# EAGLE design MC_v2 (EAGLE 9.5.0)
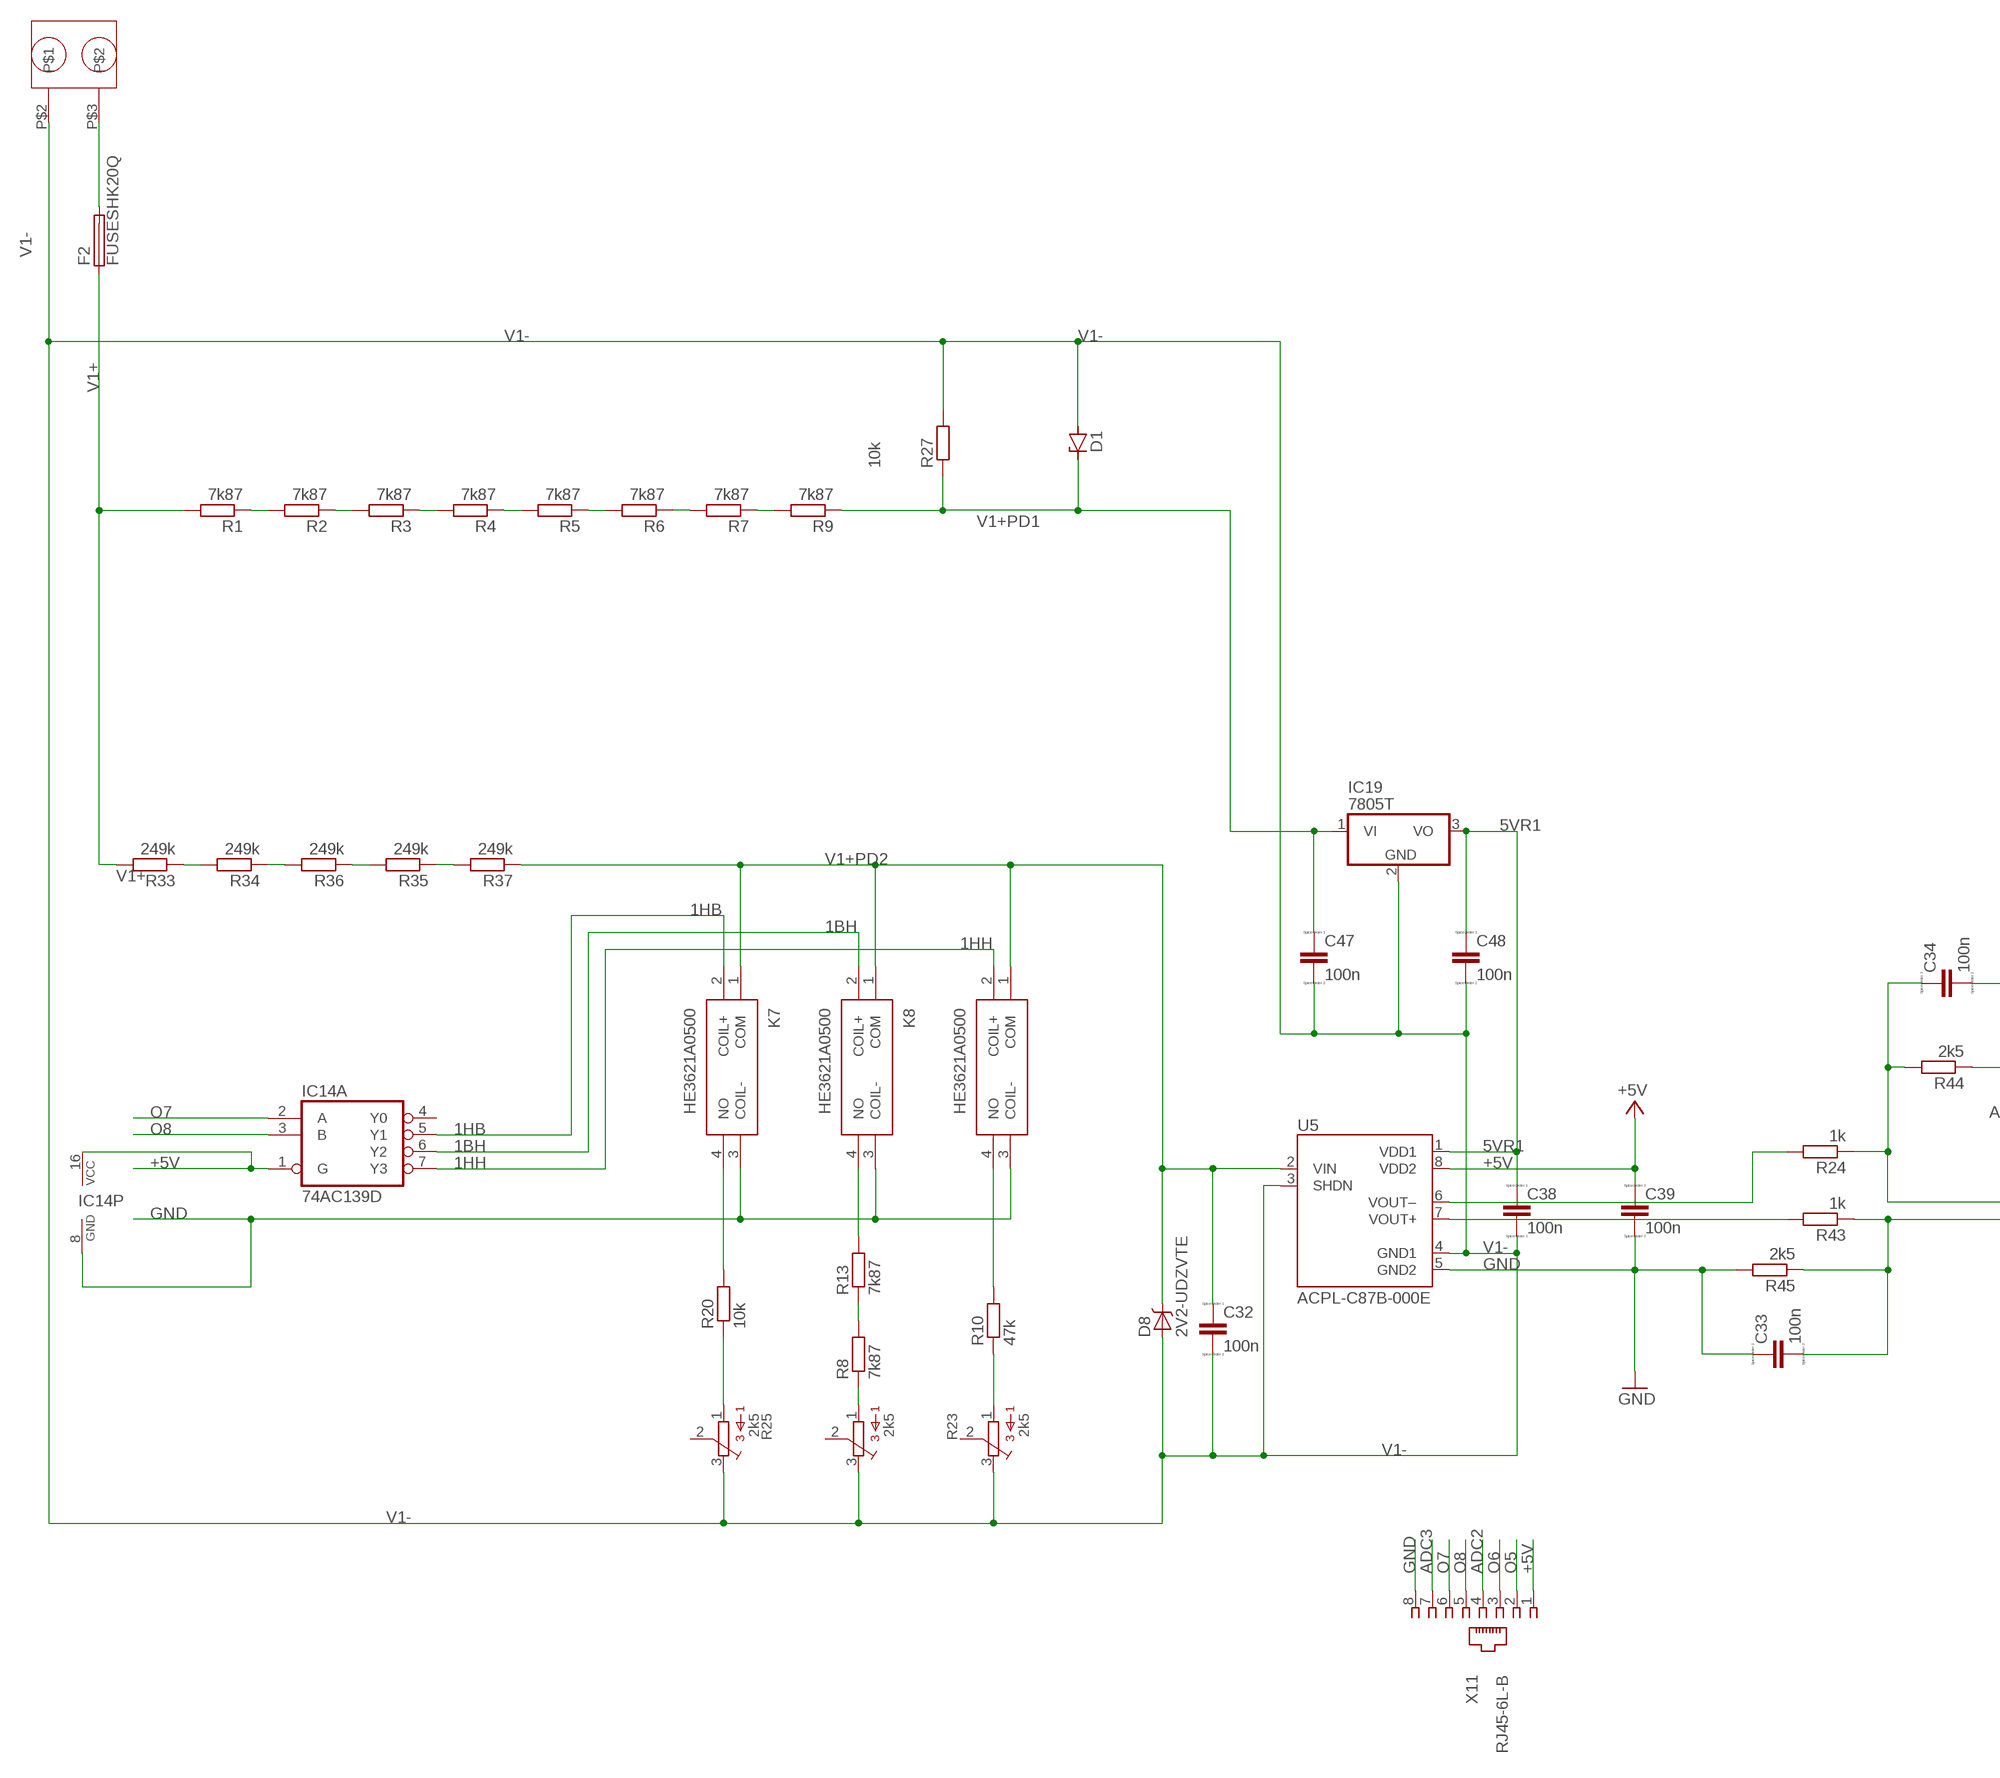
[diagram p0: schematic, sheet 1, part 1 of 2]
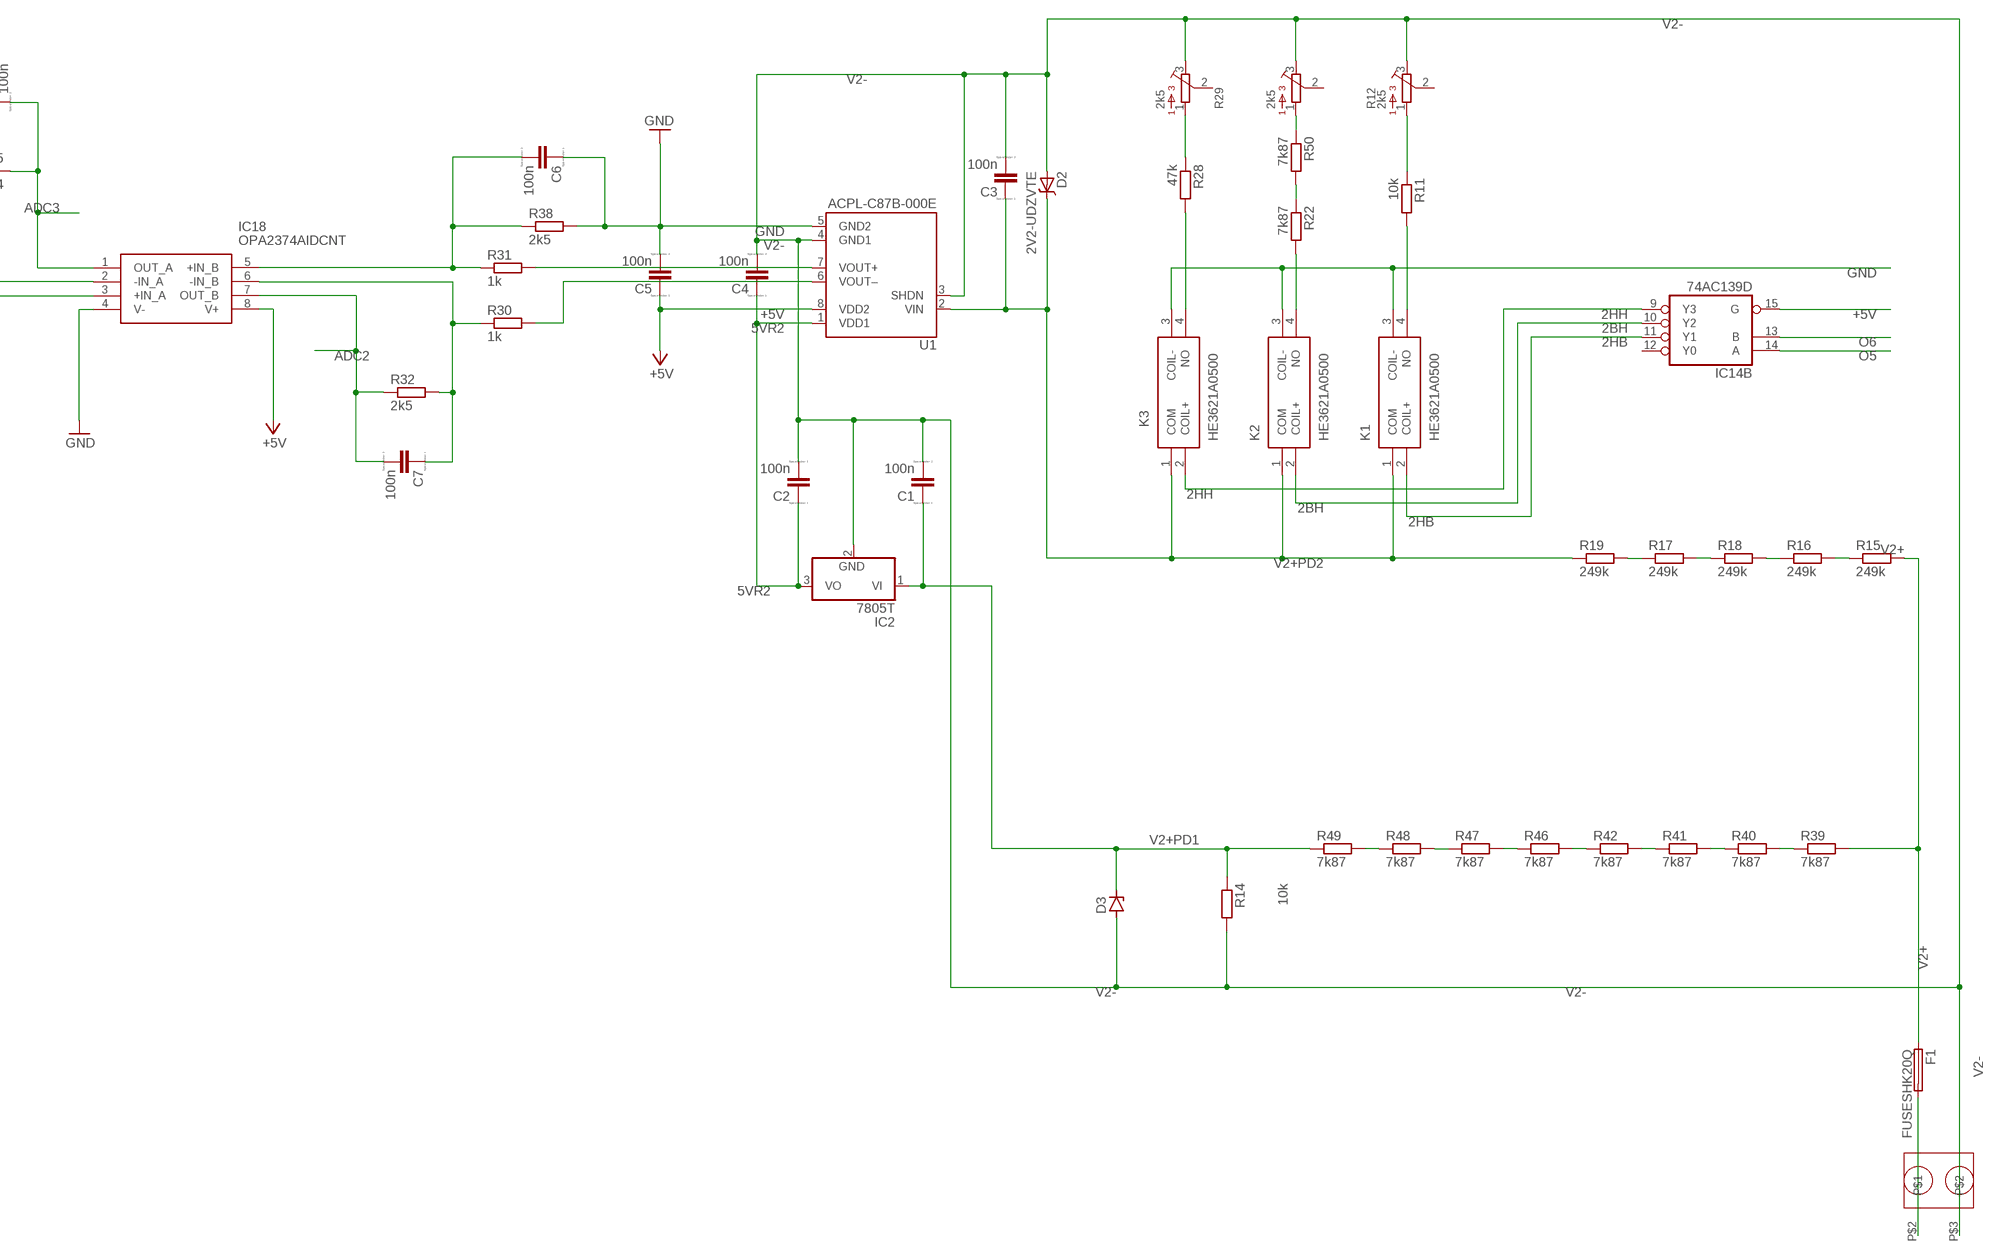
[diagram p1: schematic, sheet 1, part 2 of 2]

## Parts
C1  100n  CC2012  [C2012]
C2  100n  CC2012  [C2012]
C3  100n  CC2012  [C2012]
C4  100n  CC2012  [C2012]
C5  100n  CC2012  [C2012]
C6  100n  CC2012  [C2012]
C7  100n  CC2012  [C2012]
C32  100n  CC2012  [C2012]
C33  100n  CC2012  [C2012]
C34  100n  CC2012  [C2012]
C38  100n  CC2012  [C2012]
C39  100n  CC2012  [C2012]
C47  100n  CC2012  [C2012]
C48  100n  CC2012  [C2012]
D1  ZENER-DIODEDO41Z10  [DO41Z10]
D2  2V2-UDZVTE  BAS70J  [SOD-323]
D3  ZENER-DIODEDO41Z10  [DO41Z10]
D8  2V2-UDZVTE  BAS70J  [SOD-323]
F1  FUSESHK20Q  [SHK20Q]
F2  FUSESHK20Q  [SHK20Q]
IC2  7805T  [TO220H]
IC14  74AC139D  [SO16]
IC18  OPA2374AIDCNT  [SOT65P280X145-8N]
IC19  7805T  [TO220H]
K1  HE3621A0500  [HE3621A0500]
K2  HE3621A0500  [HE3621A0500]
K3  HE3621A0500  [HE3621A0500]
K7  HE3621A0500  [HE3621A0500]
K8  HE3621A0500  [HE3621A0500]
K9  HE3621A0500  [HE3621A0500]
R1  7k87  R-EU_M0805  [M0805]
R2  7k87  R-EU_M0805  [M0805]
R3  7k87  R-EU_M0805  [M0805]
R4  7k87  R-EU_M0805  [M0805]
R5  7k87  R-EU_M0805  [M0805]
R6  7k87  R-EU_M0805  [M0805]
R7  7k87  R-EU_M0805  [M0805]
R8  7k87  R-EU_M0805  [M0805]
R9  7k87  R-EU_M0805  [M0805]
R10  47k  R-EU_M0805  [M0805]
R11  10k  R-EU_M0805  [M0805]
R12  2k5  3362P  [3362P]
R13  7k87  R-EU_M0805  [M0805]
R14  10k  R-EU_M0805  [M0805]
R15  249k  R-EU_M0805  [M0805]
R16  249k  R-EU_M0805  [M0805]
R17  249k  R-EU_M0805  [M0805]
R18  249k  R-EU_M0805  [M0805]
R19  249k  R-EU_M0805  [M0805]
R20  10k  R-EU_M0805  [M0805]
R21  2k5  3362P  [3362P]
R22  7k87  R-EU_M0805  [M0805]
R23  2k5  3362P  [3362P]
R24  1k  R-EU_M0805  [M0805]
R25  2k5  3362P  [3362P]
R26  2k5  3362P  [3362P]
R27  10k  R-EU_M0805  [M0805]
R28  47k  R-EU_M0805  [M0805]
R29  2k5  3362P  [3362P]
R30  1k  R-EU_M0805  [M0805]
R31  1k  R-EU_M0805  [M0805]
R32  2k5  R-EU_M0805  [M0805]
R33  249k  R-EU_M0805  [M0805]
R34  249k  R-EU_M0805  [M0805]
R35  249k  R-EU_M0805  [M0805]
R36  249k  R-EU_M0805  [M0805]
R37  249k  R-EU_M0805  [M0805]
R38  2k5  R-EU_M0805  [M0805]
R39  7k87  R-EU_M0805  [M0805]
R40  7k87  R-EU_M0805  [M0805]
R41  7k87  R-EU_M0805  [M0805]
R42  7k87  R-EU_M0805  [M0805]
R43  1k  R-EU_M0805  [M0805]
R44  2k5  R-EU_M0805  [M0805]
R45  2k5  R-EU_M0805  [M0805]
R46  7k87  R-EU_M0805  [M0805]
R47  7k87  R-EU_M0805  [M0805]
R48  7k87  R-EU_M0805  [M0805]
R49  7k87  R-EU_M0805  [M0805]
R50  7k87  R-EU_M0805  [M0805]
U1  ACPL-C87B-000E  [SOIC127P1150X360-8N]
U5  ACPL-C87B-000E  [SOIC127P1150X360-8N]
U$1  BORNIER-508  [BORNIER-508_FOOTPRINT]
U$20  BORNIER-508  [BORNIER-508_FOOTPRINT]
X11  RJ45-6L-B  [RJ45-NO-SHIELD]

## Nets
1BH: IC14.6(A:Y2) K8.2(COIL+)
1HB: IC14.5(A:Y1) K7.2(COIL+)
1HH: IC14.7(A:Y3) K9.2(COIL+)
2BH: IC14.10(B:Y2) K2.2(COIL+)
2HB: IC14.11(B:Y1) K1.2(COIL+)
2HH: IC14.9(B:Y3) K3.2(COIL+)
5VR1: C38.1 C48.1 IC19.3(VO) U5.1(VDD1)
5VR2: C2.1 C4.1 IC2.3(VO) U1.1(VDD1)
+5V [power]: C5.1 C39.1 IC14.1(A:G) IC14.15(B:G) IC14.16(P:VCC) IC18.8(V+) U1.8(VDD2) U5.8(VDD2) X11.1
ADC2: C7.2 IC18.7(OUT_B) R32.1 X11.4
ADC3: C34.2 IC18.1(OUT_A) R44.1 X11.7
GND: C5.2 C6.1 C33.1 C39.2 IC14.8(P:GND) IC18.4(V-) K1.3(COIL-) K2.3(COIL-) K3.3(COIL-) K7.3(COIL-) K8.3(COIL-) K9.3(COIL-) R38.2 R45.2 U1.5(GND2) U5.5(GND2) X11.8
N$1: F1.2A U$1.P$2
N$2: F2.2A U$20.P$3
N$3: R8.1 R21.1
N$4: R8.2 R13.1
N$5: R34.1 R36.2
N$6: R1.1 R2.2
N$7: R2.1 R3.2
N$8: R3.1 R4.2
N$9: R4.1 R5.2
N$10: R5.1 R6.2
N$11: R6.1 R7.2
N$12: R7.1 R9.2
N$13: K7.4(NO) R20.2
N$14: R35.1 R37.2
N$15: R10.1 R23.1
N$16: C6.2 IC18.5(+IN_B) R31.1 R38.1
N$17: R17.2 R18.1
N$18: K9.4(NO) R10.2
N$19: R15.1 R16.2
N$20: R31.2 U1.7(VOUT+)
N$21: R30.2 U1.6(VOUT–)
N$22: C7.1 IC18.6(-IN_B) R30.1 R32.2
N$23: R11.1 R12.1
N$24: K1.4(NO) R11.2
N$25: K2.4(NO) R22.2
N$26: K3.4(NO) R28.2
N$27: R28.1 R29.1
N$30: R26.1 R50.1
N$31: R22.1 R50.2
N$32: R39.1 R40.2
N$33: R40.1 R41.2
N$34: R41.1 R42.2
N$35: R42.1 R46.2
N$36: R46.1 R47.2
N$37: R47.1 R48.2
N$38: R48.1 R49.2
N$39: R16.1 R18.2
N$40: R17.1 R19.2
N$58: R20.1 R25.1
N$69: C33.2 IC18.3(+IN_A) R43.1 R45.1
N$73: R35.2 R36.1
N$74: R33.1 R34.2
N$82: R43.2 U5.7(VOUT+)
N$83: R24.2 U5.6(VOUT–)
N$84: C34.1 IC18.2(-IN_A) R24.1 R44.2
N$107: K8.4(NO) R13.2
O5: IC14.14(B:A) X11.2
O6: IC14.13(B:B) X11.3
O7: IC14.2(A:A) X11.6
O8: IC14.3(A:B) X11.5
V1+: F2.1A R1.2 R33.2
V1+PD1: C47.1 D1.C IC19.1(VI) R9.1 R27.1
V1+PD2: C32.1 D8.C K7.1(COM) K8.1(COM) K9.1(COM) R37.1 U5.2(VIN)
V1-: C32.2 C38.2 C47.2 C48.2 D1.A D8.A IC19.2(GND) R21.3 R23.3 R25.3 R27.2 U5.3(SHDN) U5.4(GND1) U$20.P$2
V2+: F1.1A R15.2 R39.2
V2+PD1: C1.1 D3.C IC2.1(VI) R14.1 R49.1
V2+PD2: C3.1 D2.C K1.1(COM) K2.1(COM) K3.1(COM) R19.1 U1.2(VIN)
V2-: C1.2 C2.2 C3.2 C4.2 D2.A D3.A IC2.2(GND) R12.3 R14.2 R26.3 R29.3 U1.3(SHDN) U1.4(GND1) U$1.P$3
Unconnected: IC14.4(A:Y0) IC14.12(B:Y0) R12.2 R21.2 R23.2 R25.2 R26.2 R29.2

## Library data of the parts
C1-C7 C32-C34 C38 C39 C47 C48 = eagle-ltspice:C: CAPACITOR, European symbol; SPICEMODEL: NONE; SPICEPREFIX: C
D1 D3 = diode:ZENER-DIODE: Z-Diode
D2 D8 = ELL-i-DiscreteSemi:BAS70: Silicon Schottky Diodes
F1 F2 = fuse:FUSE: Fuse; OC_FARNELL: unknown; OC_NEWARK: unknown
IC2 IC19 = linear:78*: Positive VOLTAGE REGULATOR Source: http://cache.national.com/ds/LM/LM78L05.pdf http://www.fairchildsemi.com/ds/LM/LM7805.pdf
IC14 = 74xx-eu:74*139: Dual 2-line to 4-line DECODER/DEMULTIPLEXER; SPICEPREFIX: I
IC18 = OPA2374AIDCNT:OPA2374AIDCNT: Texas Instruments OPA2374AIDCNT, Dual Op Amp, 6.5MHz CMOS, Rail to Rail, 3 V, 5 V, 8-Pin SOT-23 Source: Datasheet; DESCRIPTION: Texas Instruments OPA2374AIDCNT, Dual Op Amp, 6.5MHz CMOS, Rail to Rail, 3 V, 5 V, 8-Pin SOT-23; HEIGHT: mm; MANUFACTURER_NAME: Texas Instruments; MANUFACTURER_PART_NUMBER: OPA2374AIDCNT; MOUSER_PART_NUMBER: 595-OPA2374AIDCNT; MOUSER_PRICE-STOCK: https://www.mouser.com/Search/Refine.aspx?Keyword=595-OPA2374AIDCNT
K1-K3 K7-K9 = HE3621A0500:HE3621A0500: Reed Relays REED RELAY Source: Datasheet; DESCRIPTION: Reed Relays REED RELAY; HEIGHT: 7mm; MANUFACTURER_NAME: Hamlin / Littelfuse; MANUFACTURER_PART_NUMBER: HE3621A0500; MOUSER_PART_NUMBER: 934-HE3621A0500; MOUSER_PRICE-STOCK: https://www.mouser.com/Search/Refine.aspx?Keyword=934-HE3621A0500
R1-R11 R13-R20 R22 R24 R27 R28 R30-R50 = rcl:R-EU_: RESISTOR, European symbol; SPICEPREFIX: R
R12 R21 R23 R25 R26 R29 = bourns:3362: 3362 Series 1/4" Square Trimmer
U1 U5 = ACPL-C87B-000E:ACPL-C87B-000E: Precision Optically Isolated Voltage Sensor; AVAILABILITY: Unavailable; DESCRIPTION: Isolation Amplifier, Optically, 1, 9.9 mV, 5 kV, 3V to 5.5V, SOIC, 8; MF: Broadcom Limited; MP: ACPL-C87B-000E; PACKAGE: SO-8 Broadcom; PRICE: None
U$1 U$20 = bornier-508:BORNIER-508
X11 = con-tycoelectronics:RJ45: CORCOM Modular RJ Jacks No Shield Source: www.tycoelectronics.com .. ENG_DS_1654001_1099_RJ_L_0507.pdf; MPN: RJ45-6L-B; OC_FARNELL: unknown; OC_NEWARK: 16R6090

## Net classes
0 default: width 0.152 mm, drill 0.61 mm, clearance 0.152 mm
1 power: width 0.152 mm, drill 0.61 mm, clearance 0.152 mm
2 VIN: width 0.61 mm, drill 0.61 mm, clearance 0.254 mm

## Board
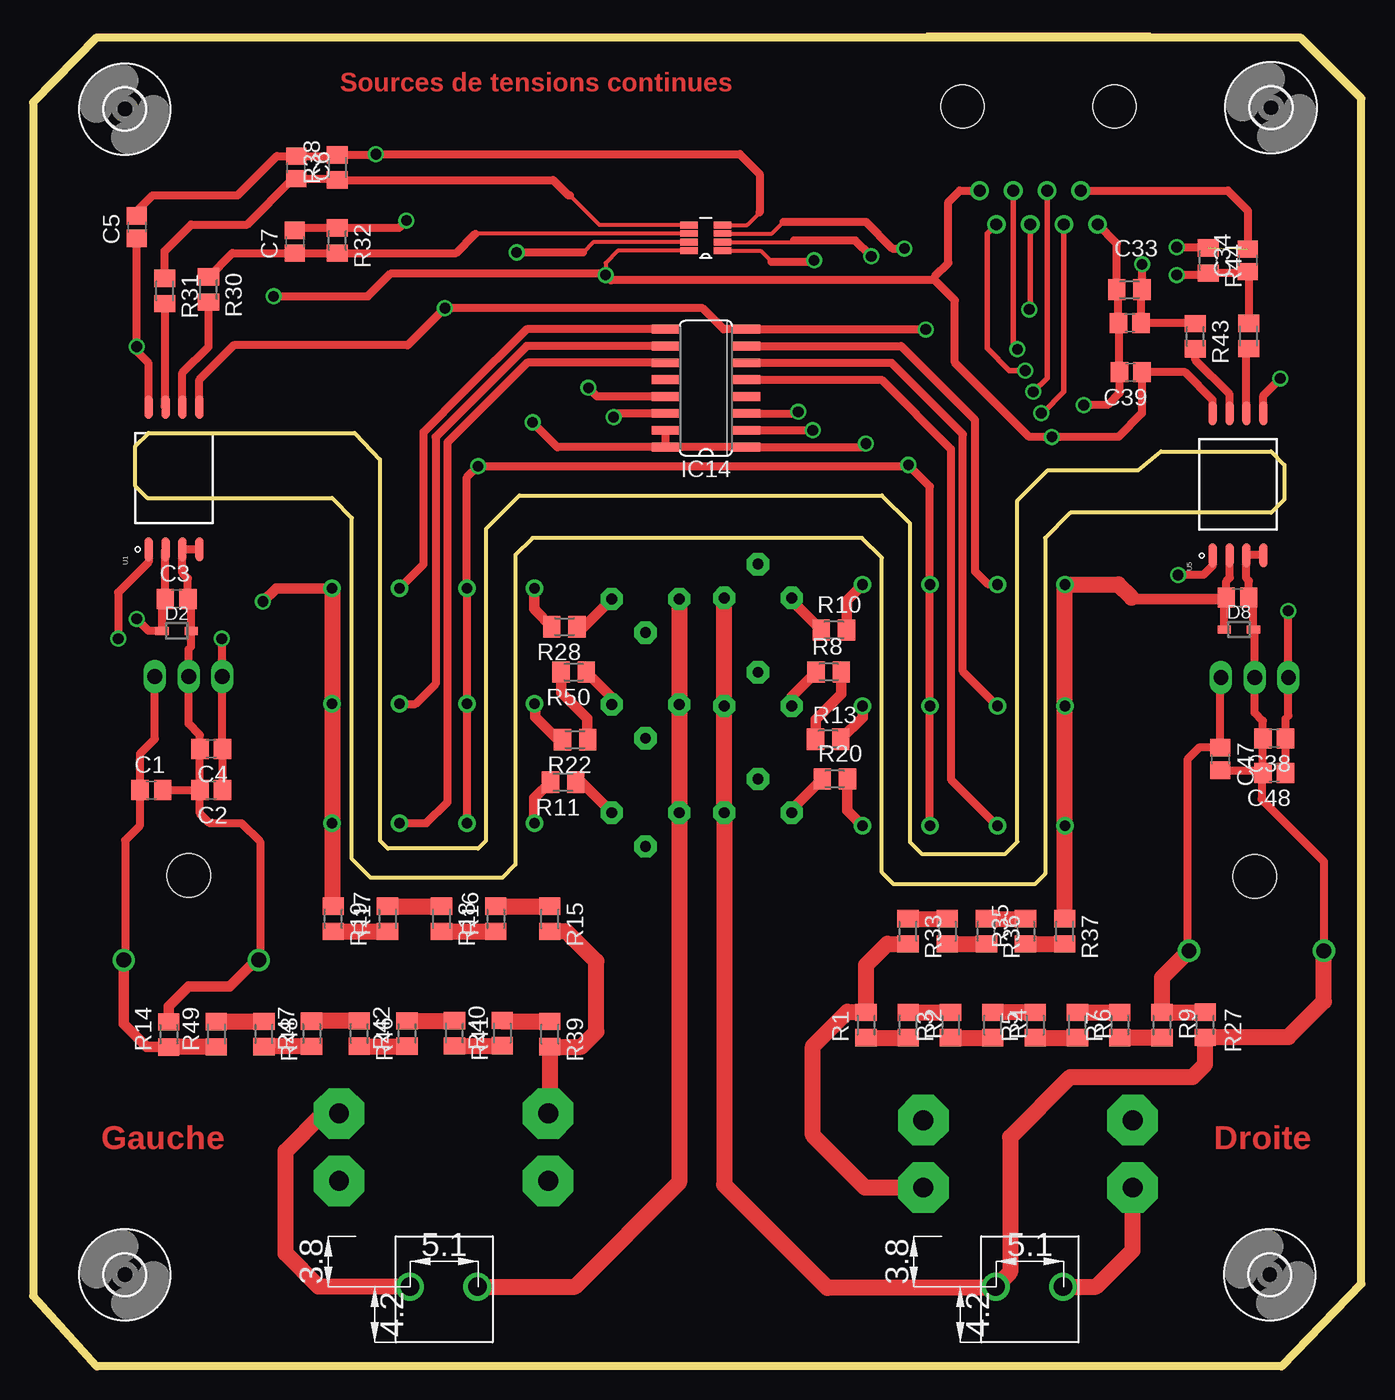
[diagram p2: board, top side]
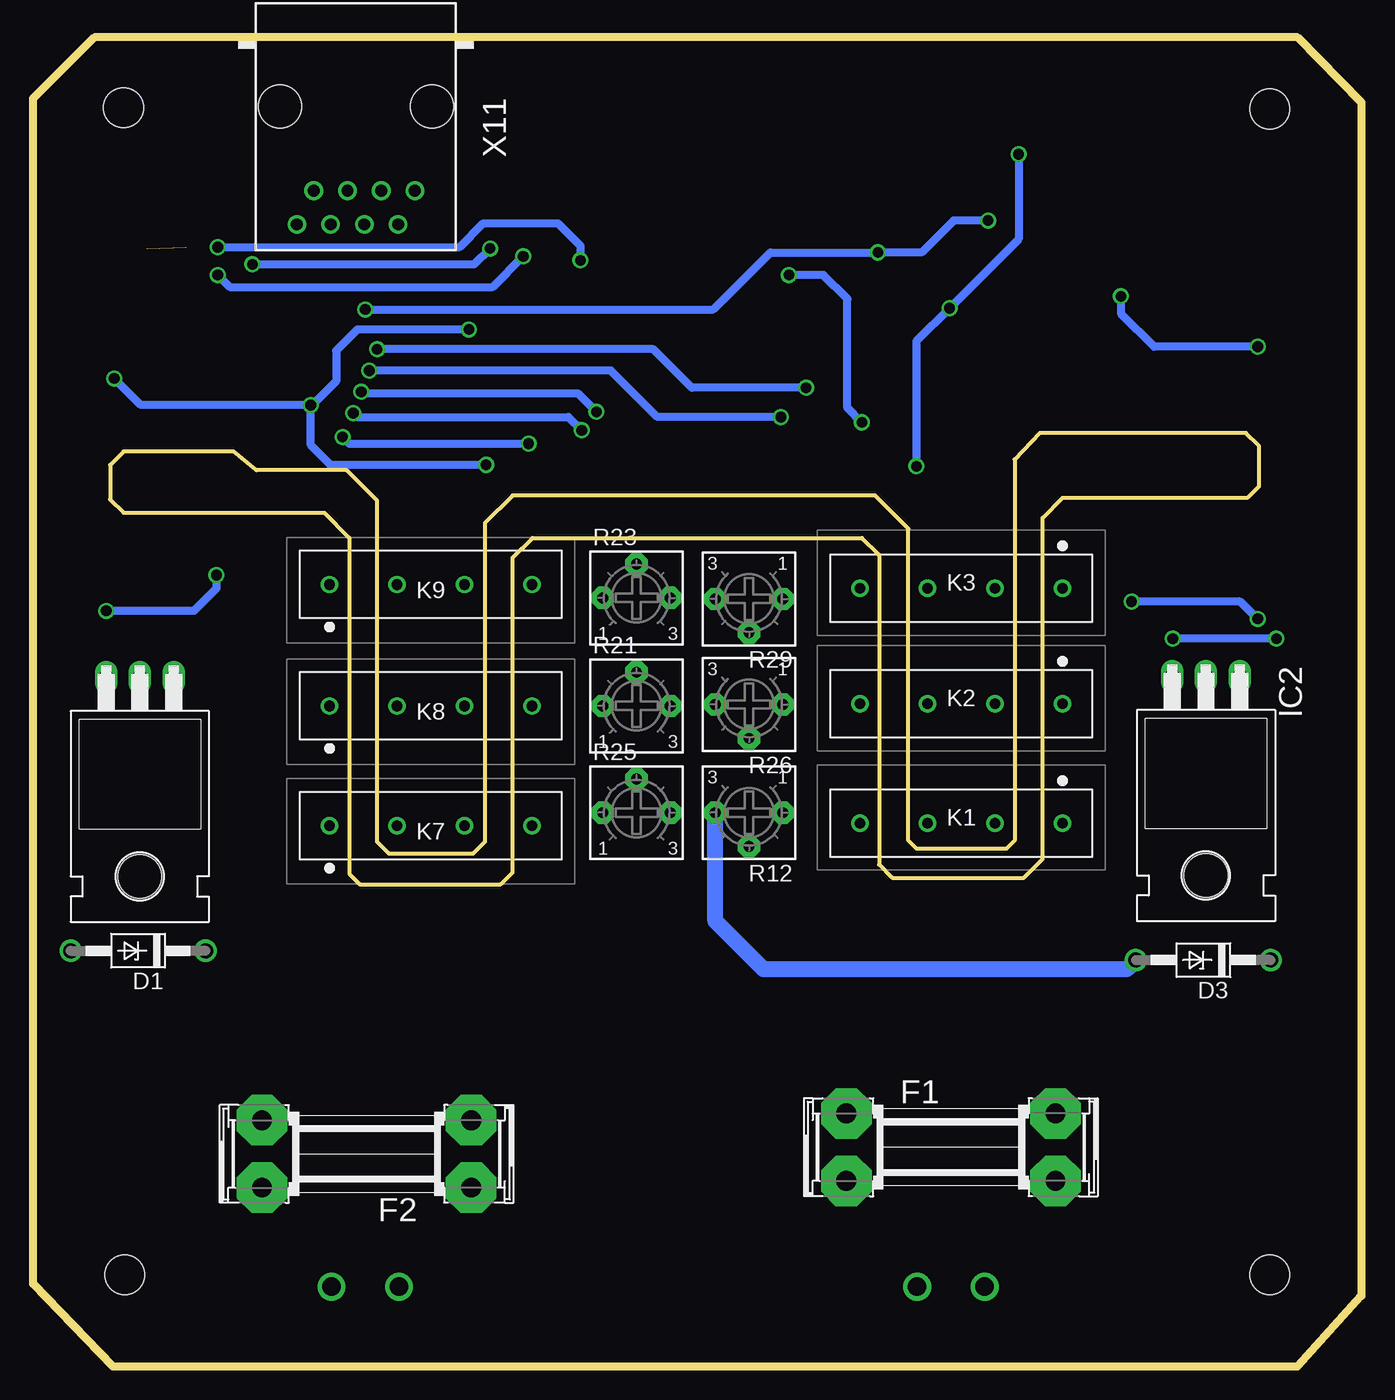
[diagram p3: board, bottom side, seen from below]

Size 100 x 100.41 mm. Coordinates in mm from the lower left corner, seen from the top.
Outline: 7.7,69.3 8.7,70.3 24.2,70.3 26.1,68.3 26.1,39.6 26.7,39 33.5,39 34.1,39.6 34.1,63.1 36.6,65.6 63.9,65.6 66,63.5 66,39.5 66.9,38.6 73.2,38.6 74.1,39.5 74.1,65.2 76.4,67.5 83.2,67.5 84.9,68.9 93.2,68.9 94.2,67.9 94.2,65.3 93.2,64.3 78.1,64.3 76.2,62.4 76.2,37.1 75.4,36.3 64.8,36.3 63.9,37.2 63.9,60.9 62.4,62.4 37.6,62.4 36.3,61.1 36.3,37.8 35.3,36.8 25.4,36.8 24,38.2 24,63.9 22.5,65.4 8.6,65.4 7.7,66.3 7.7,69.3
Outline: 4.8,0 0,5.3 0,95.2 4.8,100.1 95.4,100.1 100,95.5 100,6.2 94,0 4.8,0
Copper layers (1*16): Top 0.035mm / dielectric 1.5mm / Bottom 0.035mm
Design rules "ArduinoETH *": minimum track width 0.2mm, minimum drill 0.8mm, track to track 0.3mm, track to pad 0.3mm, pad to pad 0.2mm, via to via 0.2mm, smd to smd 0.3mm, copper to edge 25mil, drill to drill 10mil, minimum pad ring 10mil, minimum via ring 8mil, stop-mask expansion 1mil, vias tented up to drill 30mil, thermal gap 10mil

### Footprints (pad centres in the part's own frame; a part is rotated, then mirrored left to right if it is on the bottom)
C2012 = smd 1.3 x 1.5: 1 -0.85,0; 2 0.85,0
DO41Z10 = drill 1.118: A 5.08,0; C -5.08,0
SOD-323 = smd 1 x 0.6: A 1.1,0; C -1.1,0
SHK20Q = drill 1.5 pad 3.81 octagon: 1A -7.874,2.54; 1B -7.874,-2.54; 2A 7.874,2.54; 2B 7.874,-2.54
TO220H = drill 1.118 long: 1 -2.54,-10.16; 2 0,-10.16; 3 2.54,-10.16 | hole 3.302: 0,4.826
SO16 = smd 0.66 x 2.032: 1 -4.445,-3.073; 2 -3.175,-3.073; 3 -1.905,-3.073; 4 -0.635,-3.073; 5 0.635,-3.073; 6 1.905,-3.073; 7 3.175,-3.073; 8 4.445,-3.073; 9 4.445,3.073; 10 3.175,3.073; 11 1.905,3.073; 12 0.635,3.073; 13 -0.635,3.073; 14 -1.905,3.073; 15 -3.175,3.073; 16 -4.445,3.073
SOT65P280X145-8N = smd 1.321 x 0.508: 1 -1.27,0.965; 2 -1.27,0.33; 3 -1.27,-0.33; 4 -1.27,-0.965; 5 1.27,-0.965; 6 1.27,-0.33; 7 1.27,0.33; 8 1.27,0.965
HE3621A0500 = drill 0.8 pad 1.3: 1 0,0; 2 5.08,0; 3 10.16,0; 4 15.24,0
M0805 = smd 1.3 x 1.6: 1 -0.95,0; 2 0.95,0
3362P = drill 0.813 pad 1.676 octagon: 1 -2.54,0; 2 0,2.54; 3 2.54,0
SOIC127P1150X360-8N = smd 1.8 x 0.6: 1 -5.35,1.905; 2 -5.35,0.635; 3 -5.35,-0.635; 4 -5.35,-1.905; 5 5.35,-1.905; 6 5.35,-0.635; 7 5.35,0.635; 8 5.35,1.905
BORNIER-508_FOOTPRINT = drill 1.4: P$2 -0.04,0; P$3 5.04,0
3,0 = hole 3: 0,0
RJ45-NO-SHIELD = drill 0.9 pad 1.4: 1 -4.445,6.35; 2 -3.175,8.89; 3 -1.905,6.35; 4 -0.635,8.89; 5 0.635,6.35; 6 1.905,8.89; 7 3.175,6.35; 8 4.445,8.89 | hole 3.251: -5.715,0; 5.715,0

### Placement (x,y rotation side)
C1  8.9,43.4 0 top
C2  13.4,43.4 180 top
C3  10.8,57.8 0 top
C4  13.4,46.5 180 top
C5  7.8,85.8 90 top
C6  19.8,90.3 270 top
C7  19.7,84.7 90 top
C32  90.68,57.89 0 top
C33  82.57,78.58 0 top
C34  91.46,83.3 90 top
C38  93.44,47.29 180 top
C39  82.63,74.88 180 top
C47  89.39,45.74 270 top
C48  93.44,44.7 180 top
D1  92.1,31.3 180 bottom
D2  10.8,55.4 0 top
D3  11.9,30.6 180 bottom
D8  90.78,55.5 0 top
F1  30.9,16.5 0 bottom
F2  74.9,16 180 bottom
IC2  11.7,41.8 180 bottom
IC14  50.66,73.68 90 top
IC18  50.64,84.99 180 top
IC19  91.97,41.73 180 bottom
K1  22.5,40.91 180 bottom
K2  22.5,49.9 180 bottom
K3  22.5,58.6 180 bottom
K7  77.68,40.72 0 bottom
K8  77.68,49.74 0 bottom
K9  77.68,58.89 0 bottom
R1  62.7,25.7 90 top
R2  65.89,25.7 270 top
R3  69.07,25.7 90 top
R4  72.26,25.7 270 top
R5  75.44,25.7 90 top
R6  78.63,25.7 270 top
R7  81.81,25.7 90 top
R8  59.9,52.3 0 top
R9  85,25.7 270 top
R10  60.29,55.46 0 top
R11  39.9,44 180 top
R12  46.1,41.7 180 bottom
R13  59.85,47.24 0 top
R14  10.2,25 90 top
R15  38.9,33.7 270 top
R16  34.83,33.7 90 top
R17  26.67,33.7 90 top
R18  30.75,33.7 270 top
R19  22.6,33.7 270 top
R20  60.35,44.24 0 top
R21  54.57,49.74 0 bottom
R22  40.8,47.2 180 top
R23  54.57,57.88 0 bottom
R24  91.52,77.6 270 top
R25  54.57,41.7 0 bottom
R26  46.1,49.85 180 bottom
R27  88.25,25.72 270 top
R28  40,55.7 180 top
R29  46.1,57.8 180 bottom
R30  13.2,81.1 270 top
R31  9.9,81 270 top
R32  22.9,84.8 270 top
R33  65.87,32.77 270 top
R34  68.82,32.77 90 top
R35  74.72,32.77 90 top
R36  71.77,32.77 270 top
R37  77.67,32.77 270 top
R38  22.9,90.3 90 top
R39  38.9,25.03 270 top
R40  35.31,25.1 90 top
R41  31.72,25.09 270 top
R42  28.14,25.08 90 top
R43  87.5,77.58 270 top
R44  88.47,83.3 270 top
R45  82.54,81.1 180 top
R46  24.55,25.06 270 top
R47  20.96,25.05 90 top
R48  17.37,25.04 270 top
R49  13.79,25.01 90 top
R50  40.7,52.3 180 top
U1  10.6,66.9 90 top
U5  90.71,66.44 90 top
U$1  28.4,6 0 top
U$2  [3,0]  6.9,94.7 90 top
U$3  [3,0]  93.2,94.8 90 top
U$6  [3,0]  93.1,6.9 90 top
U$7  [3,0]  6.9,6.9 90 top
U$20  72.5,6 0 top
X11  75.7,94.9 180 bottom

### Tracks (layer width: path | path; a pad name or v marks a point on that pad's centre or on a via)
1BH
  Top 0.6: IC14.6 64.62,75.58 70,70.2 70,52.34 K8.2
1HB
  Top 0.6: IC14.5 63.89,74.31 69.1,69.1 69.1,44.22 K7.2
1HH
  Top 0.6: IC14.7 65.35,76.85 70.9,71.3 70.9,59.9 71.91,58.89 K9.2
2BH
  Top 0.6: K2.2 28.8,49.9 30.3,51.4 30.3,70 37.15,76.85 IC14.10
2HB
  Top 0.6: K1.2 29.61,40.91 31.2,42.5 31.2,69.6 37.18,75.58 IC14.11
2HH
  Top 0.6: K3.2 29.4,60.42 29.4,70.37 32.5,73.47 | 32.5,73.47 32.5,73.5 | IC14.9 37.15,78.12 32.5,73.47
5VR1  (via drill 0.8)
  Top 0.6: v94.5,56.9 94.51,56.89 IC19.3 94.51,49.01 94.29,48.79 C38.1 C48.1 | U5.1 88.81,60.31 88.1,59.6 v86.2,59.6 86.1,59.6
  Bottom 0.6: v86.2,59.6 86.2,58.6 87.9,56.9 v94.5,56.9
5VR2  (via drill 0.8)
  Top 0.6: C2.1 C4.1 IC2.3 14.24,54.76 v14.2,54.8 | U1.1 8.7,60.6 6.4,58.3 v6.4,54.8
  Bottom 0.6: v6.4,54.8 v14.2,54.8
+5V  (via drill 0.8)
  Top 0.3: IC18.8 44.03,84.03 43.1,83.1 v43.1,82.2
  Top 0.6: IC14.16 IC14.1 62.43,69.23 v62.7,69.5 | U1.8 8.7,75.55 7.8,76.45 v7.8,76.8 C5.1 | IC14.15 IC14.16 | IC14.16 39.47,69.23 v37.6,71.1 | U5.8 88.81,72.79 86.72,74.88 C39.1 83.48,71.78 81.7,70 v76.7,70 75,70 69.4,75.6 69.4,80.3 67.9,81.8 | X11.1 69.75,88.55 68.9,87.7 68.9,83.1 67.9,82.1 67.9,81.8 | 67.9,81.8 43.5,81.8 v43.1,82.2 43,82.3 26.9,82.3 25.2,80.6 v18.1,80.6
  Bottom 0.6: v7.8,76.8 15.6,76.8 18.1,79.3 v18.1,80.6 18.2,80.6 | v37.6,71.1 38.7,72.2 38.7,80.4 40.5,82.2 v43.1,82.2 | v62.7,69.5 76.2,69.5 v76.7,70
ADC2  (via drill 0.8)
  Top 0.3: IC18.7 42.17,84.67 41.4,83.9
  Top 0.4: X11.4 75.06,79.67 v75,79.6
  Top 0.6: C7.2 19.9,85.75 R32.1 27.55,85.75 v28.1,86.3 | 41.4,83.9 v36.4,83.9
  Bottom 0.6: v75,79.6 48.8,79.6 44.5,83.9 v36.4,83.9 33.1,83.9 30.7,86.3 v28.1,86.3
ADC3  (via drill 0.8)  (1 unrouted)
  Top 0.3: IC18.1 54.77,84.03 55.6,83.2
  Top 0.6: R44.1 86.15,84.25 v86.1,84.3 | X11.7 89.95,88.55 91.46,87.04 C34.2 | 55.6,83.2 58.7,83.2 v58.8,83.3
  Bottom 0.6: v86.1,84.3 67.9,84.3 66.1,86.1 60.5,86.1 58.8,84.4 v58.8,83.3
GND  (via drill 0.8)
  Top 0.3: IC18.4 53.76,85.96 54.7,86.9
  Top 0.6: 67.62,40.62 K7.3 K8.3 K9.3 67.52,66.28 v65.9,67.9 65.8,67.8 v33.5,67.8 32.66,66.96 K3.3 K2.3 K1.3 | U1.5 12.51,74.3 15.1,76.9 28.2,76.9 v31,79.7 50.4,79.7 51.98,78.12 IC14.8 67.18,78.12 v67.2,78.1 | X11.8 81.59,84.57 R45.2 81.72,80.97 C33.1 81.78,78.52 C39.2 81.78,73.28 80.9,72.4 v79.1,72.4 79,72.4 | U5.5 92.62,73.12 v93.9,74.4 | C5.2 7.8,87 9,88.2 15.4,88.2 18.35,91.15 C6.1 22.8,91.15 R38.2 25.75,91.25 v25.8,91.3 53.2,91.3 54.7,89.8 54.7,86.9
  Bottom 0.6: v79.1,72.4 91.9,72.4 v93.9,74.4 | v25.8,91.3 25.8,84.9 v31,79.7 33.5,77.2 v33.5,67.8 33.5,67.6 | v67.2,78.1 75.6,78.1 77.2,76.5 77.2,74.2 79,72.4 v79.1,72.4 | v65.9,67.9 77.6,67.9 79.1,69.4 v79.1,72.4
N$1
  Top 1.2: U$1.P$2 21.5,6 19,8.5 19,16.2 21.84,19.04 F1.2A
N$2
  Top 1.2: U$20.P$3 80.04,6 82.77,8.73 F2.2A
N$3
  Top 0.8: R21.1 57.11,50.46 R8.1
N$4
  Top 0.8: R13.1 58.9,48.7 60.85,50.65 R8.2
N$5
  Top 1.2: R34.1 R36.2
N$6
  Top 1.2: R1.1 R2.2
N$7
  Top 1.2: R2.1 R3.2
N$8
  Top 1.2: R3.1 R4.2
N$9
  Top 1.2: R5.2 R4.1
N$10
  Top 1.2: R5.1 R6.2
N$11
  Top 1.2: R6.1 R7.2
N$12
  Top 1.2: R9.2 R7.1
N$13
  Top 0.8: K7.4 61.3,41.86 R20.2
N$14
  Top 1.2: R35.1 R37.2
N$15
  Top 0.8: R10.1 57.11,57.69 R23.1
N$16
  Top 0.3: IC18.5 42.64,85.96 40.4,88.2
  Top 0.6: 40.4,88.2 40.3,88.2 39.15,89.35 R38.1 22.8,89.45 C6.2 19.55,89.45 16.1,86 11.9,86 9.9,84 R31.1
N$17
  Top 1.2: R17.2 R18.1
N$18
  Top 0.8: R10.2 61.24,57.68 K9.4
N$19
  Top 1.2: R16.2 R15.1
N$20
  Top 0.6: R31.2 9.9,72.32 U1.7
N$21
  Top 0.6: U1.6 11.23,74.83 13.2,76.8 R30.2
N$22
  Top 0.3: IC18.6 33.33,85.33 33.3,85.3
  Top 0.6: R30.1 15,83.85 C7.1 R32.2 31.85,83.85 33.3,85.3
N$23
  Top 0.8: R11.1 41.26,44 R12.1
N$24
  Top 0.8: K1.4 37.74,42.79 R11.2
N$25
  Top 0.8: K2.4 37.8,49.84 37.8,48.9 39.5,47.2 R22.2
N$26
  Top 0.8: K3.4 37.74,57.06 37.8,57 37.8,56.95 R28.2
N$27
  Top 0.8: R28.1 41.46,55.7 R29.1
N$30
  Top 0.8: R50.1 43.56,50.39 R26.1
N$31
  Top 0.8: R22.1 41.7,47.25 41.7,48.8 39.75,50.75 R50.2
N$32
  Top 1.2: R40.2 35.39,25.98 R39.1
N$33
  Top 1.2: R41.2 35.3,24.14 R40.1
N$34
  Top 1.2: R42.2 31.71,26.03 R41.1
N$35
  Top 1.2: R46.2 28.12,24.11 R42.1
N$36
  Top 1.2: R46.1 R47.2
N$37
  Top 1.2: R47.1 20.95,24.09 R48.2
N$38
  Top 1.2: R49.2 17.35,25.96 R48.1
N$39
  Top 1.2: R18.2 R16.1
N$40
  Top 1.2: R19.2 R17.1
N$58
  Top 0.8: R25.1 57.11,41.95 R20.1
N$69  (via drill 0.8)
  Top 0.3: IC18.3 55.62,85.33 56.5,86.2
  Top 0.6: R43.1 87.44,78.58 C33.2 83.42,81.02 R45.1 83.49,82.99 v83.5,83 | 56.5,86.2 62.7,86.2 64.7,84.2 v65.6,84.2
  Bottom 0.6: v83.5,83 66.8,83 v65.6,84.2
N$73
  Top 1.2: R36.1 R35.2
N$74
  Top 1.2: R33.1 R34.2
N$82
  Top 0.6: U5.7 90.08,73.22 87.5,75.8 R43.2
N$83
  Top 0.6: R24.2 91.35,76.49 U5.6
N$84  (via drill 0.8)
  Top 0.3: IC18.2 57.17,84.67 57.3,84.8
  Top 0.6: R24.1 91.52,82.39 C34.1 91.36,82.35 R44.2 88.33,82.2 v86.1,82.2 | 57.3,84.8 61.9,84.8 v63.1,83.6
  Bottom 0.6: v86.1,82.2 85.2,81.3 65.4,81.3 v63.1,83.6
N$107
  Top 0.8: R13.2 62.44,48.88 K8.4
O5  (via drill 0.8)
  Top 0.4: X11.2 71.83,85.31 71.83,76.67 73.5,75 v74.7,75
  Top 0.6: IC14.14 43.97,71.77 v43.7,71.5
  Bottom 0.6: v43.7,71.5 53,71.5 56.5,75 v74.7,75
O6  (via drill 0.8)
  Top 0.4: v74.1,76.6 73.8,76.91 X11.3
  Top 0.6: IC14.13 42.46,73.04 v41.8,73.7
  Bottom 0.6: v41.8,73.7 50.4,73.7 53.3,76.6 v74.1,76.6
O7  (via drill 0.8)
  Top 0.4: v75.9,71.8 76,71.8 77.61,73.41 X11.6
  Top 0.6: v58.7,70.5 IC14.2
  Bottom 0.6: v75.9,71.8 75.6,71.5 59.7,71.5 v58.7,70.5
O8  (via drill 0.8)
  Top 0.4: v75.3,73.4 76.34,74.44 X11.5
  Top 0.6: IC14.3 57.47,71.77 v57.6,71.9
  Bottom 0.6: v75.3,73.4 75.2,73.3 59,73.3 v57.6,71.9
V1+
  Top 1.2: R33.2 64.32,31.82 62.7,30.2 R1.2 62.65,26.7 61.3,26.7 58.7,24.1 58.7,17.4 62.64,13.46 F2.1A
V1+PD1
  Top 0.6: IC19.1 89.39,51.85 C47.1 87.79,46.59 86.9,45.7 86.9,31.42 D1.C
  Top 1.2: R27.1 88.23,26.65 R9.1 85,29.28 D1.C
V1+PD2
  Top 0.6: C32.1 89.83,59.13 90.1,59.4 90.1,61.07 U5.2 | D8.C 89.68,57.74 C32.1 | C32.1 89.73,57.8
  Top 0.8: 89.73,57.8 82.81,57.8 82.7,57.9
  Top 1.2: R37.1 77.68,33.73 K7.1 K8.1 K9.1 81.71,58.89 82.7,57.9
V1-
  Top 0.6: U5.4 U5.3 91.35,59.35 91.53,59.17 C32.2 91.88,57.55 D8.A 91.97,55.41 IC19.2 91.97,49.23 92.59,48.61 C38.2 C48.2 | C47.2 92.4,44.89 C48.2 | C48.2 92.5,44.61 92.5,42.7 97.18,38.02 D1.A
  Top 1.2: R23.3 R21.3 R25.3 52.03,13.67 59.8,5.9 72.36,5.9 U$20.P$2 73.56,7.1 73.56,17.26 78.1,21.8 87.3,21.8 88.25,22.75 R27.2 88.28,24.8 94.5,24.8 97.18,27.48 D1.A
V2+
  Top 1.2: R15.2 | F1.1A 38.9,19.17 R39.2 41.28,24.08 42.4,25.2 42.4,30.5 40.15,32.75 R15.2
V2+PD1
  Top 0.6: D3.C 6.92,30.7 6.92,39.62 8.05,40.75 C1.1 8.05,46.15 9.16,47.26 IC2.1
  Top 0.8: R14.1 8.55,24.05 6.82,25.78 D3.C
  Top 1.2: R49.1 10.21,24.06 R14.1
V2+PD2  (via drill 0.8)
  Top 0.6: U1.2 9.95,61.54 C3.1 9.7,57.55 D2.C 8.7,55.4 v7.8,56.3
  Top 0.8: K3.1 18.3,58.6 v17.3,57.6
  Top 1.2: K3.1 K2.1 K1.1 22.5,34.75 R19.1
  Bottom 0.6: v7.8,56.3 9.1,57.6 v17.3,57.6
V2-
  Top 0.6: C1.2 C2.2 | C2.2 C4.2 12.55,47.55 11.7,48.4 IC2.2 11.7,54 11.9,54.2 D2.A 11.9,57.55 C3.2 11.65,59.35 11.23,59.77 U1.3 U1.4 | D3.A 17.08,30.7 17.08,39.52 15.7,40.9 13.3,40.9 12.55,41.65 C2.2
  Top 0.8: D3.A 16.8,30.6 14.8,28.6 11.7,28.6 10.2,27.1 R14.2
  Top 1.2: R29.3 R26.3 R12.3 48.64,13.84 40.8,6 U$1.P$3
  Bottom 1.2: D3.A 17.68,29.9 45,29.9 48.64,33.54 R12.3

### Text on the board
Top: Sources de tensions continues | Gauche | Droite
